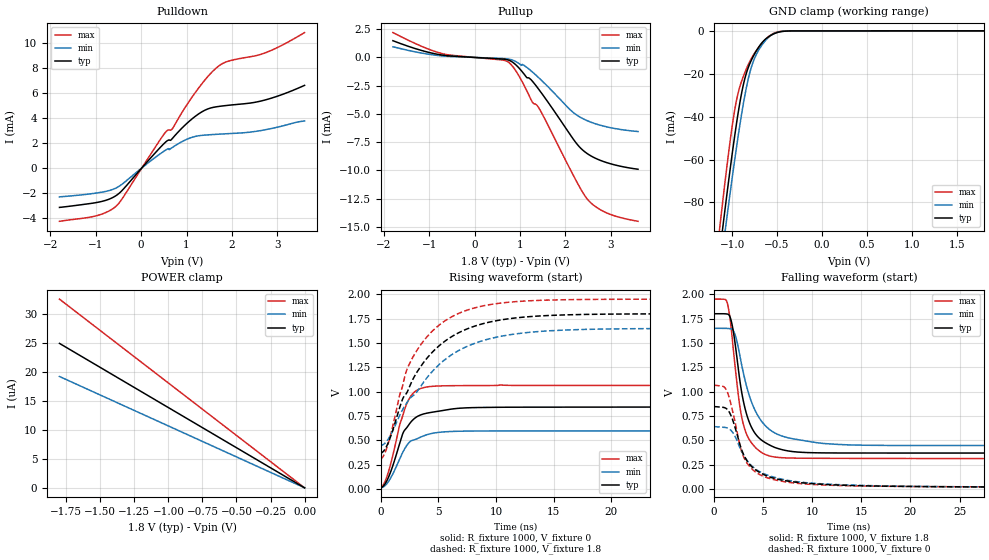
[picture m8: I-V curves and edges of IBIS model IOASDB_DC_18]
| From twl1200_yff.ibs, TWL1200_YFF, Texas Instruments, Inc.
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[Model]   IOASDB_DC_18
Model_type  I/O
Vinl=0.63
Vinh=1.17
Enable   Active-Low
Vref =   1.8
Rref =   1M
Cref =   15p
Vmeas =   0.9
| variable   typ   min   max
C_comp   4.20pF   3.56pF   5.01pF
| C_pullup   4.18pF   3.55pF   4.78pF
| C_pulldown   4.51pF   3.74pF   5.23pF
| C_tri-state   4.20pF   3.56pF   5.01pF
[Temperature Range]   40   100   -40
| Ambient temperature   25   85   -40
[Voltage range]   1.8   1.65   1.95
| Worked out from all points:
|   slope of the pulldown table from 0 to 0.27 V, typ, clamps not added: 244 ohm
|   slope of the pullup table from 0 to 0.27 V, typ, clamps not added: 4.38 kohm
|   GND clamp passes 1 mA (typ) near -0.51 V on its own axis
|   rising waveform, R_fixture 1000, V_fixture 0: 20-80 % time 1.69ns typ, 1.64ns min, 1.4ns max; typ from 0.013 V to 0.847 V
|   falling waveform, R_fixture 1000, V_fixture 1.8: 20-80 % time 1.6ns typ, 2.35ns min, 1.28ns max; typ from 1.8 V to 0.369 V
|   rising waveform, R_fixture 1000, V_fixture 1.8: 20-80 % time 4.34ns typ, 5.19ns min, 3.45ns max; typ from 0.368 V to 1.8 V
|   falling waveform, R_fixture 1000, V_fixture 0: 20-80 % time 2.49ns typ, 3.33ns min, 1.91ns max; typ from 0.847 V to 0.014 V
[GND Clamp]
| IOASDB_DC_18
|   Voltage   I(typ)   I(min)   I(max)
-1.8V     -350.5mA   -347.3mA   -356.7mA
-1.14V    -104.2mA   -113.8mA   -92.69mA
-1.125V   -99.04mA   -108.9mA   -87.15mA
-1.095V   -88.75mA   -99.02mA   -76.27mA
-1.065V   -78.65mA   -89.31mA   -65.72mA
-955mV    -44.37mA   -55.5mA    -33.26mA
-900mV    -30.34mA   -40.32mA   -24.22mA
-850mV    -21.02mA   -28.36mA   -18.63mA
-795mV    -14.55mA   -18.29mA   -13.61mA
-735mV    -9.659mA   -11.41mA   -9.515mA
-550mV    -1.676mA   -1.638mA   -1.44mA
1.8V      421.1pA    1.603uA    -2.71uA
[POWER Clamp]
| IOASDB_DC_18
|   Voltage   I(typ)   I(min)   I(max)
-1.8V     24.89uA    19.19uA    32.51uA
-170mV    2.352uA    1.816uA    3.071uA
-60mV     832.8nA    647.8nA    1.086uA
0V        0A         0A         0A
[Pulldown]
| IOASDB_DC_18
|   Voltage   I(typ)   I(min)   I(max)
-1.8V     -3.146mA   -2.301mA   -4.257mA
-970mV    -2.746mA   -1.986mA   -3.799mA
-540mV    -2.168mA   -1.567mA   -3.003mA
435mV     1.71mA     1.186mA    2.362mA
580mV     2.203mA    1.528mA    3.023mA
690mV     2.385mA    1.658mA    3.163mA
1V        3.558mA    2.298mA    5.032mA
1.27V     4.35mA     2.591mA    6.432mA
1.695V    4.93mA     2.713mA    8.135mA
1.945V    5.038mA    2.763mA    8.587mA
2.66V     5.388mA    3.021mA    9.134mA
3.6V      6.624mA    3.782mA    10.85mA
[Pullup]
| IOASDB_DC_18
|   Voltage   I(typ)   I(min)   I(max)
-1.8V     1.482mA    937.7uA    2.202mA
-720mV    211.8uA    136.5uA    344.3uA
750mV     -237uA     -143.1uA   -434uA
960mV     -861.3uA   -493.2uA   -1.521mA
1.145V    -1.76mA    -868.3uA   -2.911mA
1.285V    -2.162mA   -1.332mA   -4.02mA
1.445V    -2.997mA   -1.92mA    -4.678mA
2.135V    -7.005mA   -4.739mA   -10.13mA
2.305V    -7.899mA   -5.239mA   -11.41mA
2.48V     -8.507mA   -5.597mA   -12.52mA
2.91V     -9.308mA   -6.144mA   -13.76mA
3.6V      -9.895mA   -6.557mA   -14.5mA
[Ramp]
| IOASDB_DC_18
| variable   typ   min   max
dV/dt_r   0.50/1.69E-09   0.36/1.65E-09   0.63/1.40E-09
dV/dt_f   0.86/1.60E-09   0.72/2.35E-09   0.98/1.28E-09
R_load = 1000
[Rising Waveform]
| IOASDB_DC_18
R_fixture =   1000
C_fixture =   0
L_fixture =   0
V_fixture =   0
V_fixture_min = 0
V_fixture_max = 0
|   Time   V(typ)   V(min)   V(max)
0s        13.03mV    11.14mV    16.26mV
265ps     34.04mV    23.35mV    49.58mV
595ps     98.25mV    63.13mV    145.5mV
1.665ns   473.2mV    312mV      663.9mV
1.985ns   586mV      391.7mV    781.1mV
2.48ns    665.6mV    479.7mV    927.2mV
3.35ns    754.6mV    526.1mV    1.027V
5.06ns    799.5mV    581.6mV    1.058V
12.82ns   840.1mV    596.3mV    1.063V
240ns     846.7mV    610.8mV    1.065V
[Falling Waveform]
| IOASDB_DC_18
R_fixture =   1000
C_fixture =   0
L_fixture =   0
V_fixture =   1.8
V_fixture_min = 1.65
V_fixture_max = 1.95
|   Time   V(typ)   V(min)   V(max)
0s        1.8V       1.65V      1.95V
1.375ns   1.796V     1.649V     1.897V
1.885ns   1.659V     1.636V     1.507V
2.6ns     1.131V     1.381V     863.2mV
3.31ns    767.9mV    1.054V     562.8mV
3.935ns   609.6mV    862mV      457.9mV
4.74ns    509.6mV    709.2mV    381.6mV
6.835ns   406.4mV    546.6mV    322mV
17.65ns   369.6mV    447.7mV    313.7mV
240ns     368.6mV    446.8mV    309.7mV
[Rising Waveform]
| IOASDB_DC_18
R_fixture =   1000
C_fixture =   0
L_fixture =   0
V_fixture =   1.8
V_fixture_min = 1.65
V_fixture_max = 1.95
|   Time   V(typ)   V(min)   V(max)
0s        368.3mV    446.7mV    309.3mV
650ps     473.1mV    511.4mV    465mV
1.885ns   918.2mV    810.5mV    1.051V
2.305ns   996.7mV    892.6mV    1.235V
3.04ns    1.179V     983.7mV    1.404V
4.155ns   1.363V     1.163V     1.581V
7.455ns   1.642V     1.462V     1.835V
12.45ns   1.766V     1.604V     1.93V
27.49ns   1.799V     1.649V     1.95V
240ns     1.8V       1.65V      1.95V
[Falling Waveform]
| IOASDB_DC_18
R_fixture =   1000
C_fixture =   0
L_fixture =   0
V_fixture =   0
V_fixture_min = 0
V_fixture_max = 0
|   Time   V(typ)   V(min)   V(max)
0s        846.7mV    640.5mV    1.065V
920ps     838.5mV    634.1mV    1.053V
1.29ns    822.3mV    628.3mV    1.008V
1.85ns    720.8mV    586.3mV    813mV
2.815ns   400.8mV    383mV      381.8mV
3.93ns    220.2mV    228.9mV    198.5mV
6.365ns   103.3mV    114mV      90.02mV
10.94ns   48.78mV    53.57mV    42.26mV
41.99ns   17.55mV    16.98mV    19.96mV
240ns     13.65mV    11.9mV     16.8mV
